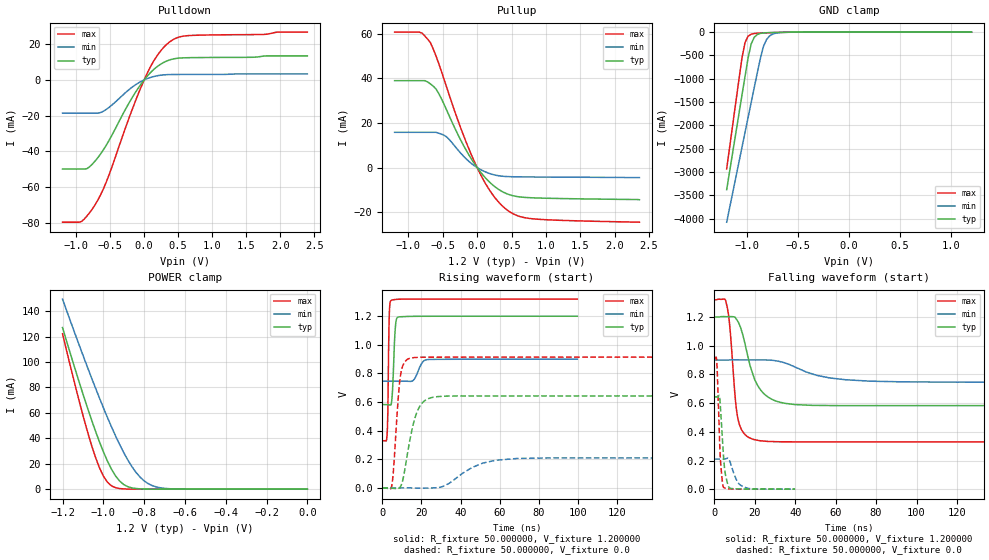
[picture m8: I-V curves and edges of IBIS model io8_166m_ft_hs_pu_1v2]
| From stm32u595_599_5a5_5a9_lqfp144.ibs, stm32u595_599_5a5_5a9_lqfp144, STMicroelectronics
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|   Model io8_166m_ft_hs_pu_1v2
[Model]  io8_166m_ft_hs_pu_1v2
Model_type I/O
Polarity   Non-Inverting
Enable   Active-Low
Vinl =   0.360000V
Vinh =   0.840000V
Vmeas =  0.600000V
Cref =   50.000000pF
Rref =   100.000000M
Vref =   0.0V
C_comp   3.151500pF   3.086800pF   3.197700pF
[Temperature Range]   25.000000   0.140000k   -40.000000
[Pullup Reference]   1.200000V   0.900000V   1.320000V
[Pulldown Reference]   0.0V   0.0V   0.0V
[POWER Clamp Reference]   1.200000V   0.900000V   1.320000V
[GND Clamp Reference]   0.0V   0.0V   0.0V
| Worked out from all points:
|   slope of the pulldown table from 0 to 0.18 V, typ, clamps not added: 25.4 ohm
|   slope of the pullup table from 0 to 0.18 V, typ, clamps not added: 27.8 ohm
|   GND clamp passes 1 mA (typ) near -0.51 V on its own axis
|   POWER clamp passes 1 mA (typ) near -0.86 V on its own axis
|   rising waveform, R_fixture 50.000000, V_fixture 1.200000: 20-80 % time 1.13ns typ, 3.03ns min, 581ps max; typ from 0.583 V to 1.2 V
|   rising waveform, R_fixture 50.000000, V_fixture 0.0: 20-80 % time 5.79ns typ, 15.2ns min, 2.79ns max; typ from 0 V to 0.643 V
|   falling waveform, R_fixture 50.000000, V_fixture 1.200000: 20-80 % time 8.14ns typ, 19.5ns min, 3.49ns max; typ from 1.2 V to 0.583 V
|   falling waveform, R_fixture 50.000000, V_fixture 0.0: 20-80 % time 1.94ns typ, 3.6ns min, 1.46ns max; typ from 0.643 V to 0 V
[Pulldown]
|Voltage   I(typ)   I(min)   I(max)
-1.2V     -49.86mA   -18.57mA   -79.56mA
-920mV    -49.86mA   -18.57mA   -79.19mA
-840mV    -49.6mA    -18.57mA   -76.08mA
-720mV    -45.32mA   -18.57mA   -69.74mA
-560mV    -36.71mA   -16.58mA   -57.44mA
-200mV    -11.43mA   -4.74mA    -19.03mA
0V        0A         0A         0A
160mV     6.477mA    2.075mA    11.78mA
360mV     10.99mA    2.99mA     20.81mA
480mV     12.07mA    3.054mA    23.52mA
640mV     12.43mA    3.075mA    24.76mA
2.4V      13.45mA    3.36mA     26.76mA
[Pullup]
|Voltage   I(typ)   I(min)   I(max)
-1.2V     38.94mA    15.8mA     60.71mA
-840mV    38.94mA    15.8mA     60.71mA
-680mV    37.5mA     15.8mA     56mA
-560mV    33.31mA    15.44mA    46.78mA
-440mV    25.54mA    13.66mA    35.67mA
-240mV    12.39mA    6.512mA    17.85mA
-40mV     1.772mA    818.2uA    2.67mA
200mV     -7.072mA   -2.851mA   -11mA
440mV     -11.84mA   -4.03mA    -19.1mA
600mV     -13.07mA   -4.154mA   -21.71mA
840mV     -13.59mA   -4.223mA   -23.04mA
2.36V     -14.4mA    -4.5mA     -24.47mA
[GND_clamp]
|Voltage   I(typ)   I(min)   I(max)
-1.2V     -3.379A    -4.076A    -2.932A
-1.05V    -1.35A     -2.47A     -550.7mA
-1.02V    -947.8mA   -2.149A    -221.5mA
-990mV    -552.4mA   -1.829A    -88.44mA
-960mV    -255.3mA   -1.51A     -44.87mA
-930mV    -111.8mA   -1.191A    -30.68mA
-870mV    -28.36mA   -564.6mA   -21.34mA
-840mV    -18.65mA   -309.5mA   -18.49mA
-810mV    -14.07mA   -161.6mA   -15.92mA
-780mV    -11.37mA   -83.33mA   -13.53mA
-600mV    -3.009mA   -4.322mA   -3.091mA
1.2V      0A         13.65nA    0A
[POWER_clamp]
|Voltage   I(typ)   I(min)   I(max)
-1.2V     127mA      149.4mA    122.2mA
-1.12V    84.98mA    114mA      70.29mA
-1.06V    55.52mA    88.42mA    35.69mA
-1.02V    37.64mA    72.04mA    17.19mA
-1V       29.52mA    64.13mA    10.33mA
-960mV    15.7mA     48.99mA    2.596mA
-900mV    3.636mA    28.77mA    207.8uA
-840mV    502.9uA    13.24mA    43.45uA
-800mV    129uA      6.535mA    43.45uA
-740mV    26.2uA     1.726mA    43.45uA
-620mV    25.1uA     82.33uA    35.72uA
0V        0A         17.36nA    0A
[Ramp]
| variable   typ   min   max
dV/dt_r  0.38570/5.78450n   0.12565/15.14921n   0.54819/2.78122n
dV/dt_f  0.37043/8.12728n   92.37000m/19.48986n 0.59404/3.47900n
R_load = 50.000000
[Rising Waveform]
R_fixture= 50.000000
V_fixture= 1.200000
V_fixture_min= 0.900000
V_fixture_max= 1.320000
|time   V(typ)   V(min)   V(max)
0s        582.6mV    746mV      329.9mV
2.402ns   582.7mV    746mV      369mV
2.803ns   582.7mV    746mV      530mV
3.203ns   582.3mV    746mV      977mV
3.604ns   581.1mV    746mV      1.236V
4.404ns   581.2mV    746mV      1.309V
6.607ns   1.115V     746.1mV    1.317V
8.008ns   1.194V     746.1mV    1.319V
23.02ns   1.2V       897.1mV    1.32V
99.7ns    1.2V       900mV      1.32V
[Rising Waveform]
R_fixture= 50.000000
V_fixture= 0.0
V_fixture_min= 0.0
V_fixture_max= 0.0
|time   V(typ)   V(min)   V(max)
0s        435.6uV    496.7uV    380uV
4.805ns   -1.1mV     496.4uV    14.8mV
5.606ns   -2.802mV   496.3uV    110.4mV
9.209ns   8.008mV    495.3uV    779.6mV
11.21ns   106.6mV    501.9uV    876.3mV
14.01ns   331.7mV    533uV      905.8mV
19.22ns   572.1mV    -783.9uV   913.1mV
28.03ns   637.9mV    2.359mV    913.9mV
58.06ns   643.2mV    193.8mV    914mV
199.4ns   643.3mV    210mV      914mV
[Falling Waveform]
R_fixture= 50.000000
V_fixture= 1.200000
V_fixture_min= 0.900000
V_fixture_max= 1.320000
|time   V(typ)   V(min)   V(max)
0s        1.2V       900mV      1.32V
5.606ns   1.202V     899.9mV    1.313V
7.608ns   1.203V     900.7mV    1.132V
10.41ns   1.194V     901.2mV    616.2mV
11.61ns   1.168V     901.2mV    492mV
19.22ns   792.6mV    900.8mV    347.7mV
26.43ns   642.9mV    900.1mV    333mV
40.04ns   589.6mV    850.3mV    330.1mV
76.88ns   582.6mV    753mV      329.9mV
199.4ns   582.6mV    746mV      329.9mV
[Falling Waveform]
R_fixture= 50.000000
V_fixture= 0.0
V_fixture_min= 0.0
V_fixture_max= 0.0
|time   V(typ)   V(min)   V(max)
0s        643.3mV    210mV      914mV
1.201ns   643.1mV    210mV      875.9mV
2.563ns   643mV      210mV      329mV
3.443ns   464.4mV    209.9mV    120.3mV
4.484ns   232.2mV    209.7mV    14.16mV
5.445ns   102.6mV    211.4mV    6.796mV
7.688ns   6.858mV    191.5mV    2.138mV
11.61ns   2.287mV    47.09mV    827.7uV
15.38ns   1.266mV    11.6mV     553.6uV
39.88ns   435.6uV    496.7uV    380uV
